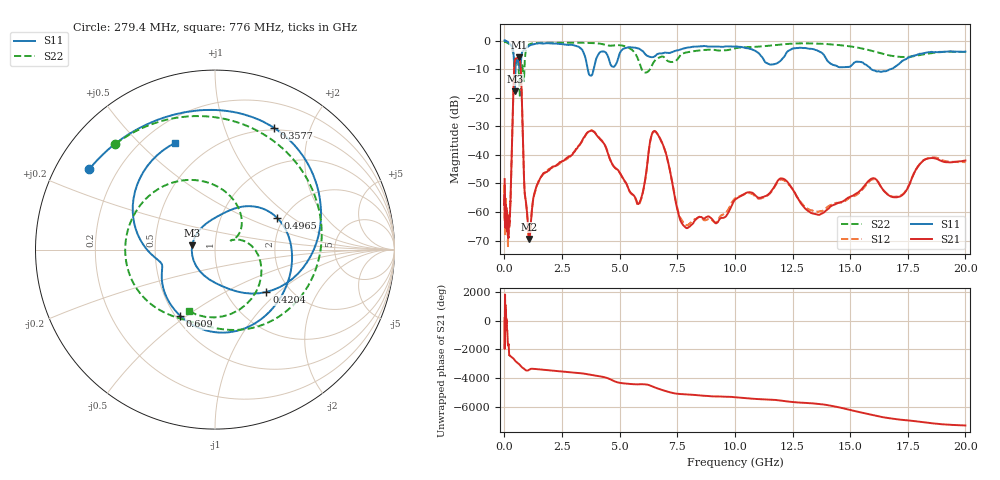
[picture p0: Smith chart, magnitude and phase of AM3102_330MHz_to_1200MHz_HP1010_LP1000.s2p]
! Date/Time: Tue, Sep 11, 2018 5:19 PM
! Network Analyzer: Agilent Technologies E8362B Rev: A.07.50.63
! Sweep from 0.010 to 20.000 GHz, 1601 Points, Sweep Type: LOG
! Power Supply: 4.949 V, 0.001 A
# Hz S DB R 50
!freq MagS11 AngS11 MagS21 AngS21 MagS12 AngS12 MagS22 AngS22
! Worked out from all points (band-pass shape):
!   1601 points, 10 MHz to 20 GHz, reference 50 ohm
!   highest |S21| = -5.81 dB at 620.7 MHz (marker M1); lowest = -69.4 dB at 1.072 GHz (marker M2)
!   |S21| within 3 dB of the highest: 432.2 MHz to 700.4 MHz (268.2 MHz wide, 47.4 % of centre)
!   lowest |S11| = -17.8 dB at 451.5 MHz (marker M3), VSWR 1.30, Z = 38.7 + j1.95 ohm
!   |S11| at or under -10 dB: 424.7 MHz to 481.5 MHz (56.8 MHz wide, 12.5 % of centre); 3.616 GHz to 3.876 GHz (259.1 MHz wide, 6.92 % of centre); 15.91 GHz to 16.76 GHz (850.5 MHz wide, 5.21 % of centre)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
!   |S22| runs from -19.9 to -0.2 dB; largest |S21 - S12| = 0.0093
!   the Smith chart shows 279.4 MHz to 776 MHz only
!   S11 on the Smith chart (normalised r, x): 279.4 MHz: 0.10, +0.29; 357.7 MHz: 0.47, +1.49; 420.4 MHz: 1.53, -0.84; 496.5 MHz: 1.86, +0.77; 609 MHz: 0.53, -0.47; 776 MHz: 0.32, +0.64
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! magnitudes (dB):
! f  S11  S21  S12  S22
! 10 MHz  0.0  -48.5  -50.9  -0.2
! 35.55 MHz  0.0  -61.5  -64.6  -0.4
! 48.64 MHz  -0.1  -59.3  -54.9  -0.5
! 126.4 MHz  -0.4  -64.4  -63.2  -0.8
! 153.6 MHz  -0.5  -63.8  -71.8  -0.9
! 279.4 MHz  -1.6  -51.6  -52.4  -1.8
! 357.7 MHz  -2.5  -27.6  -27.7  -3.6
! 420.4 MHz  -8.6  -10.7  -10.7  -6.3
! 447.2 MHz  -17.7  -7.3  -7.4  -7.4
! 451.5 MHz  -17.8  -7.1  -7.1  -7.5
! 496.5 MHz  -8.2  -6.3  -6.3  -6.3
! 609 MHz  -7.6  -5.8  -6.0  -9.0
! 620.7 MHz  -8.2  -5.8  -5.9  -10.2
! 776 MHz  -3.9  -25.4  -25.5  -8.6
! 869.7 MHz  -3.1  -51.7  -51.7  -10.1
! 1.072 GHz  -1.9  -69.4  -69.6  -1.4
! 1.59 GHz  -1.0  -47.7  -47.6  -0.8
! 3.793 GHz  -12.1  -31.5  -31.4  -0.8
! 5.652 GHz  -2.5  -54.6  -54.9  -4.3
! 6.549 GHz  -5.4  -31.7  -31.9  -6.8
! 7.92 GHz  -2.5  -65.6  -64.7  -4.1
! 20 GHz  -3.9  -42.0  -42.6  -4.0
